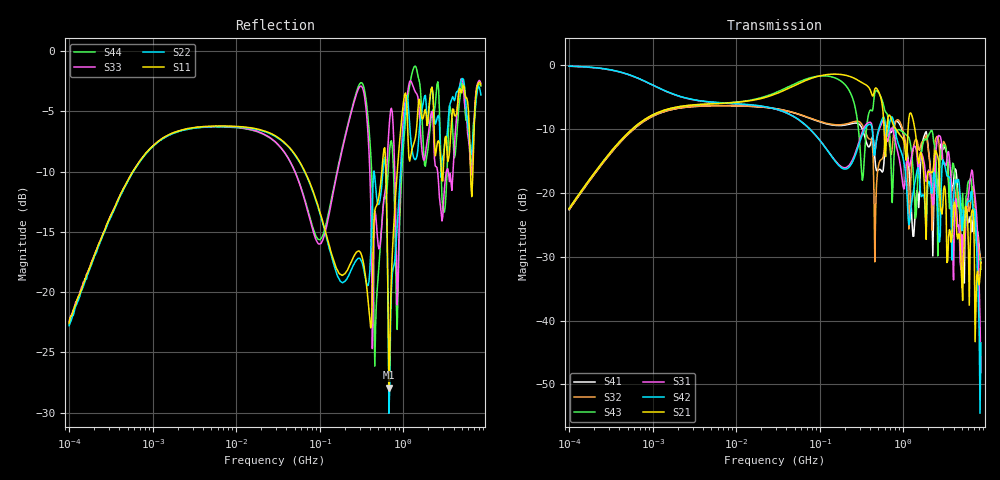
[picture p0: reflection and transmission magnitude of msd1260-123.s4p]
# MHz S MA R 50
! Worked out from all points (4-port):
!   498 points, 100 kHz to 8.5 GHz, reference 50 ohm
!   strongest paths, dB at 100 kHz, 1.698 MHz, 29.49 MHz, 500.7 MHz, 8.5 GHz:
!     S21: -22.4, -6.7, -4.5, -4.0, -30.8
!     S42: -0.1, -4.4, -6.8, -10.3, -43.5
!     S31: -0.1, -4.5, -6.9, -10.6, -48.2
!     S43: -22.4, -6.7, -4.3, -4.2, -32.0
!     S32: -22.6, -6.9, -6.8, -16.0, -30.4
!     S41: -22.6, -6.9, -6.8, -16.4, -31.0
!   lowest |S11| = -27.9 dB at 673.7 MHz (marker M1), VSWR 1.08, Z = 49.9 - j4.01 ohm
!   |S11| at or under -10 dB: 66.41 MHz to 553.4 MHz (487 MHz wide, 157 % of centre); 619.7 MHz to 847.8 MHz (228.1 MHz wide, 31.1 % of centre); 6.399 GHz to 6.814 GHz (415.2 MHz wide, 6.28 % of centre)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
0.1  0.07444 80.2  0.07549 79.6  0.9834 -4.4  0.07372 -100.4
     0.07549 79.6  0.07264 80.3  0.07401 -100.4  0.9839 -4.3
     0.9834 -4.4  0.07401 -100.4  0.07536 79.4  0.07558 79.6
     0.07372 -100.4  0.9839 -4.3  0.07558 79.6  0.07356 80.4
88.25704  0.2475 -52.4  0.8082 -3.9  0.2855 -90.1  0.3712 86.8
          0.8082 -3.9  0.245 -53.7  0.3734 85.9  0.2858 -89.2
          0.2855 -90.1  0.3734 85.9  0.1683 -21.4  0.8153 -13.3
          0.3712 86.8  0.2858 -89.2  0.8153 -13.3  0.174 -19.8
673.7244  0.04014 -88.5  0.4079 -103.4  0.2804 -63.3  0.3185 -50.8
          0.4079 -103.4  0.03145 -117.0  0.2618 -59.1  0.3282 -50.1
          0.2804 -63.3  0.2618 -59.1  0.4709 -51.4  0.3442 -159.5
          0.3185 -50.8  0.3282 -50.1  0.3442 -159.5  0.3561 -57.6
2652.059  0.4243 132.8  0.1776 19.6  0.282 101.5  0.1169 140.2
          0.1776 19.6  0.5409 127.5  0.2602 85.6  0.04894 84.4
          0.282 101.5  0.2602 85.6  0.2801 119.1  0.05742 172.5
          0.1169 140.2  0.04894 84.4  0.05742 172.5  0.694 102.2
5026.862  0.6706 -94.4  0.02071 108.9  0.04709 -120.0  0.0386 -162.6
          0.02071 108.9  0.7657 -97.2  0.01807 -144.6  0.05043 -157.6
          0.04709 -120.0  0.01807 -144.6  0.7682 -89.1  0.08077 153.7
          0.0386 -162.6  0.05043 -157.6  0.08077 153.7  0.7373 -88.4
6611.76  0.249 98.8  0.07198 25.0  0.151 48.5  0.04951 78.3
         0.07198 25.0  0.3869 74.6  0.1034 75.8  0.1034 26.5
         0.151 48.5  0.1034 75.8  0.3065 133.3  0.1141 -57.5
         0.04951 78.3  0.1034 26.5  0.1141 -57.5  0.3338 114.9
8500  0.7234 -55.6  0.02868 -22.4  0.003908 29.6  0.02829 -137.8
      0.02868 -22.4  0.6569 -59.5  0.03013 -151.0  0.00666 -70.2
      0.003908 29.6  0.03013 -151.0  0.7345 -48.3  0.02522 -32.1
      0.02829 -137.8  0.00666 -70.2  0.02522 -32.1  0.7162 -54.9
